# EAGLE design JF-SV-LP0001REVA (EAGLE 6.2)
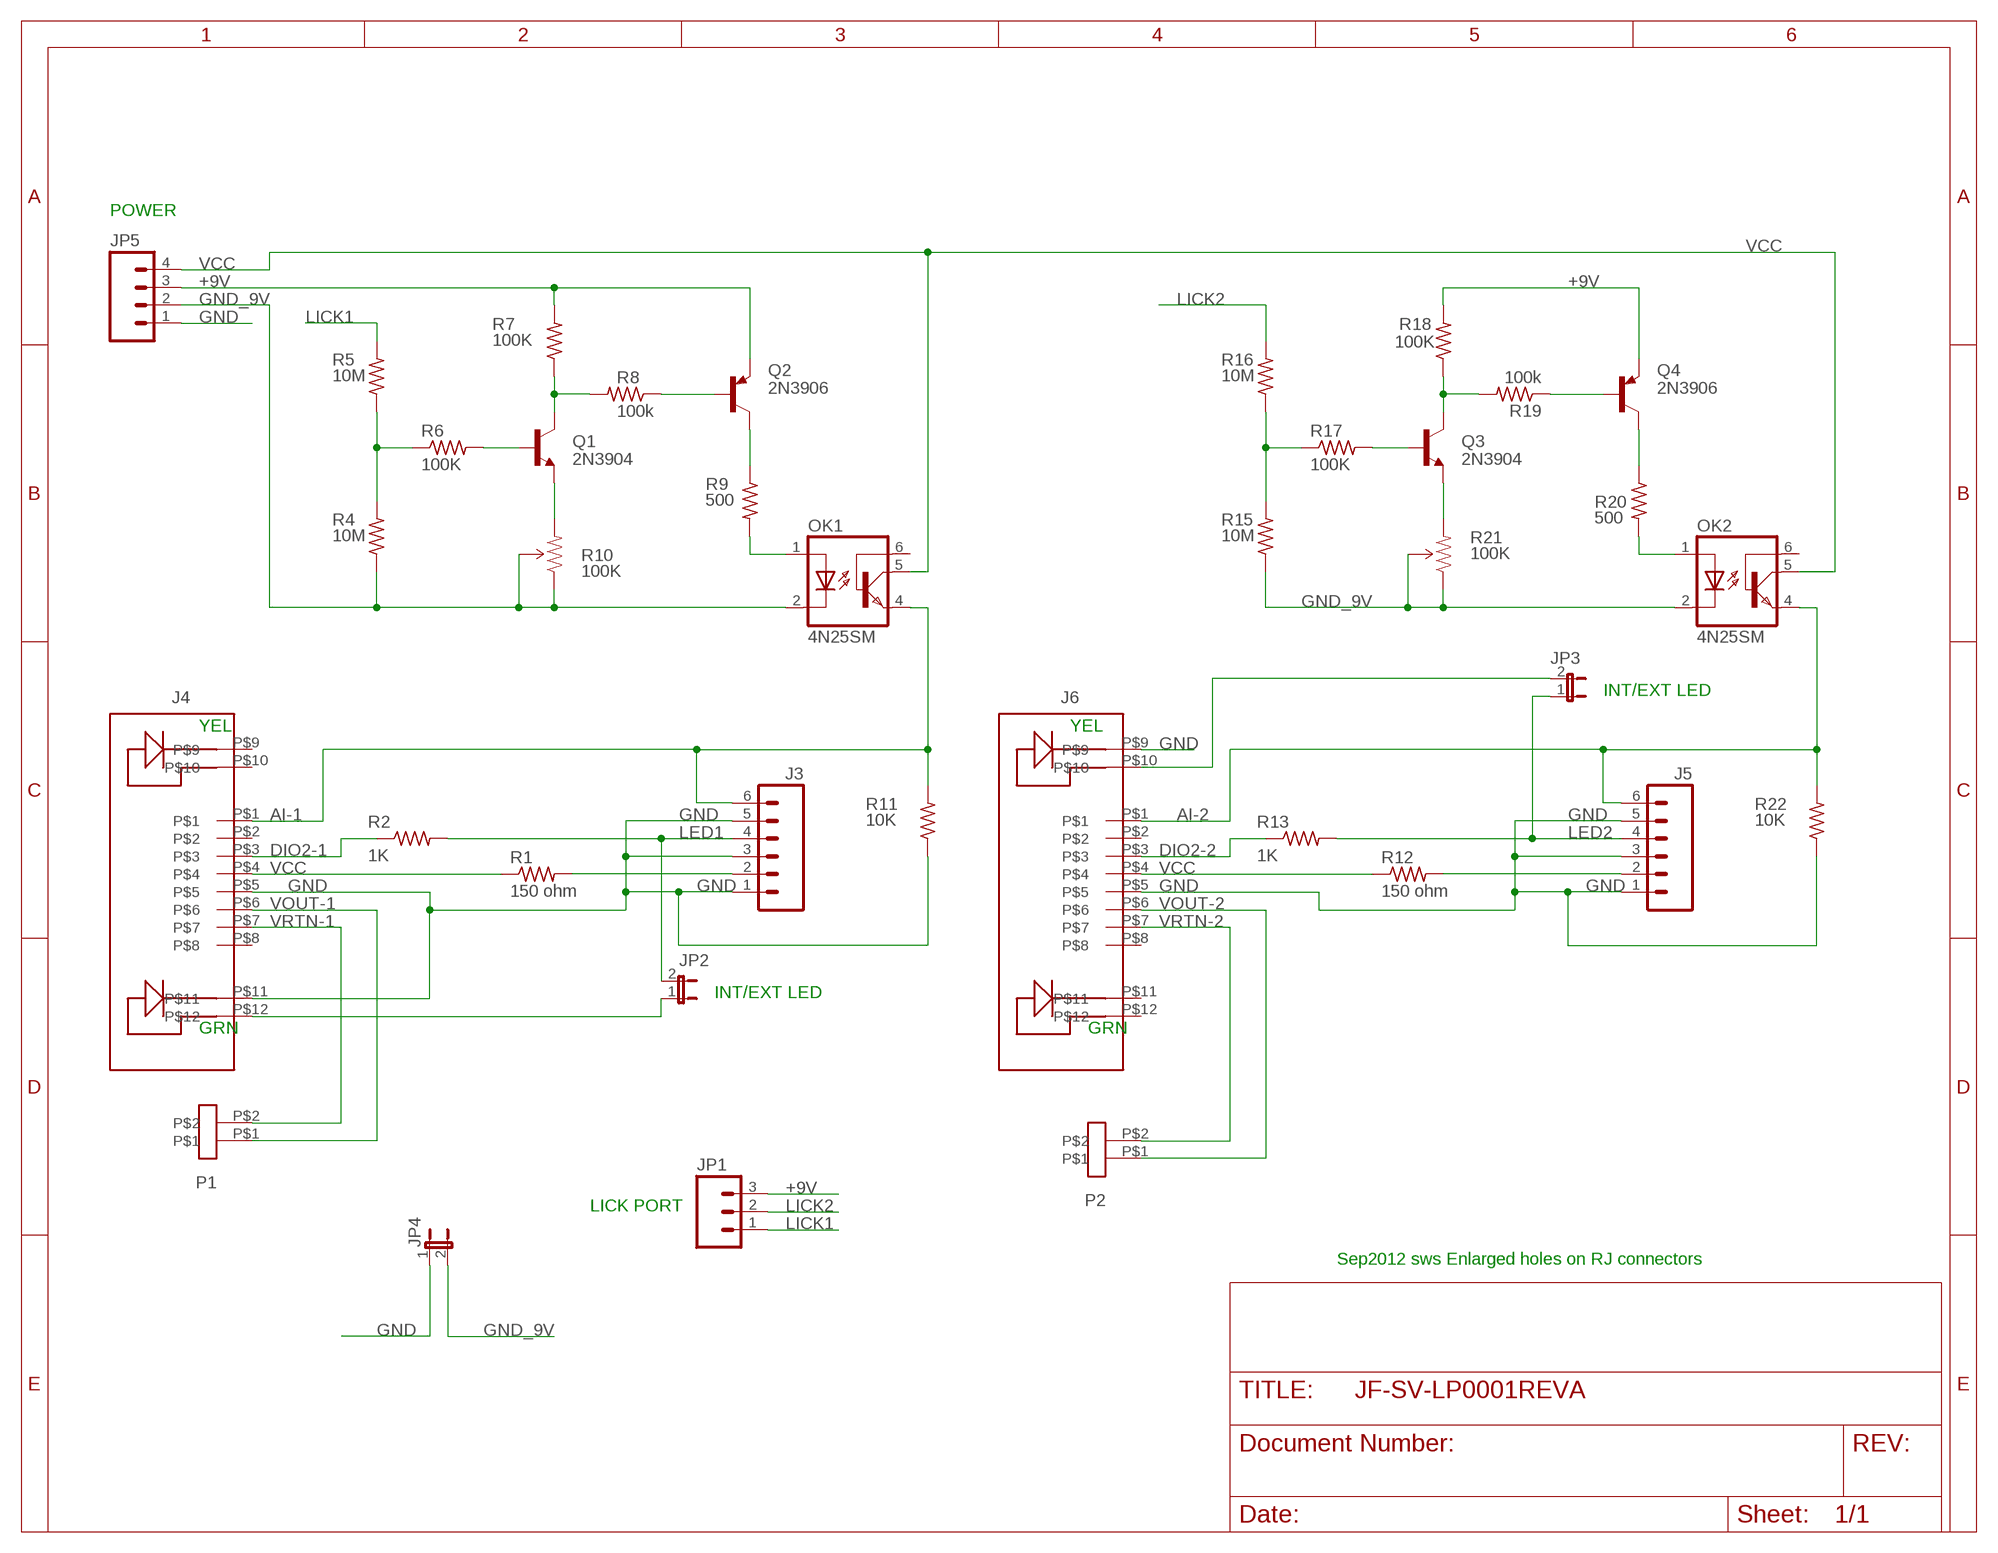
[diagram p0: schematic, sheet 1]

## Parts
J3  M063.5MM-6  [SCREWTERMINAL-3.5MM-6]
J4  RJ45_LED  [RJ45_LED]
J5  M063.5MM-6  [SCREWTERMINAL-3.5MM-6]
J6  RJ45_LED  [RJ45_LED]
JP1  M03POLAR  [MOLEX-1X3]
JP2  JP1E  [JP1]
JP3  JP1E  [JP1]
JP4  JUMPER-2PTH  [1X02]
JP5  M04POLAR  [MOLEX-1X4]
OK1  4N25SM  [DIL6-SMD]
OK2  4N25SM  [DIL6-SMD]
P1  CON2MICRO-FIT  [MICRO-FIT-2-RA]
P2  CON2MICRO-FIT  [MICRO-FIT-2-RA]
Q1  2N3904  MMBT3904LT1-NPN-SOT23-BEC  [SOT23-BEC]
Q2  2N3906  MMBT3906LT1-PNP-SOT23-BEC  [SOT23-BEC]
Q3  2N3904  MMBT3904LT1-NPN-SOT23-BEC  [SOT23-BEC]
Q4  2N3906  MMBT3906LT1-PNP-SOT23-BEC  [SOT23-BEC]
R1  150 ohm  RESISTOR_SM0805S  [0805S]
R2  1K  RESISTOR_SM0805S  [0805S]
R4  10M  RESISTOR_SM0805S  [0805S]
R5  10M  RESISTOR_SM0805S  [0805S]
R6  100K  RESISTOR_SM0805S  [0805S]
R7  100K  RESISTOR_SM0805S  [0805S]
R8  100k  RESISTOR_SM0805S  [0805S]
R9  500  RESISTOR_SM0805S  [0805S]
R10  100K  TRIMPOTPTH  [TRIM_POT_PTH]
R11  10K  RESISTOR_SM0805S  [0805S]
R12  150 ohm  RESISTOR_SM0805S  [0805S]
R13  1K  RESISTOR_SM0805S  [0805S]
R15  10M  RESISTOR_SM0805S  [0805S]
R16  10M  RESISTOR_SM0805S  [0805S]
R17  100K  RESISTOR_SM0805S  [0805S]
R18  100K  RESISTOR_SM0805S  [0805S]
R19  100k  RESISTOR_SM0805S  [0805S]
R20  500  RESISTOR_SM0805S  [0805S]
R21  100K  TRIMPOTPTH  [TRIM_POT_PTH]
R22  10K  RESISTOR_SM0805S  [0805S]

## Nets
+9V: JP1.3 JP5.3 Q2.E Q4.E R7.2 R18.2
AI-1: J3.6 J4.P$1 OK1.4(EMI) R11.2
AI-2: J5.6 J6.P$1 OK2.4(EMI) R22.2
DIO2-1: J4.P$3 R2.1
DIO2-2: J6.P$3 R13.1
GND: J3.1 J3.3 J3.5 J4.P$5 J4.P$11 J5.1 J5.3 J5.5 J6.P$5 J6.P$9 JP4.1 JP5.1 R11.1 R22.1
GND_9V: JP4.2 JP5.2 OK1.2(C) OK2.2(C) R4.1 R10.1(CCW) R10.2(WIPER) R15.1 R21.1(CCW) R21.2(WIPER)
LED1: J3.4 JP2.2 R2.2
LED2: J5.4 JP3.1 R13.2
LICK1: JP1.1 R5.2
LICK2: JP1.2 R16.2
N$1: J3.2 R1.2
N$3: OK1.1(A) R9.2
N$8: J4.P$12 JP2.1
N$12: R4.2 R5.1 R6.1
N$13: Q1.B R6.2
N$14: Q1.E R10.3(CW)
N$15: Q1.C R7.1 R8.2
N$16: Q2.B R8.1
N$18: Q2.C R9.1
N$19: J6.P$10 JP3.2
N$21: J5.2 R12.2
N$23: R15.2 R16.1 R17.1
N$24: Q3.B R17.2
N$25: Q3.E R21.3(CW)
N$26: Q3.C R18.1 R19.2
N$27: Q4.B R19.1
N$32: OK2.1(A) R20.2
N$33: Q4.C R20.1
VCC: J4.P$4 J6.P$4 JP5.4 OK1.5(COL) OK2.5(COL) R1.1 R12.1
VOUT-1: J4.P$6 P1.P$1
VOUT-2: J6.P$6 P2.P$1
VRTN-1: J4.P$7 P1.P$2
VRTN-2: J6.P$7 P2.P$2
Unconnected: J4.P$2 J4.P$8 J4.P$9 J4.P$10 J6.P$2 J6.P$8 J6.P$11 J6.P$12 OK1.6(BAS) OK2.6(BAS)

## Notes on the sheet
- POWER
- INT/EXT LED
- YEL | YEL
- INT/EXT LED
- GRN | GRN
- LICK PORT
- Sep2012 sws Enlarged holes on RJ connectors

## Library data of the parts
J3 J5 = SparkFun:M06: Header 6 Standard 6-pin 0.1" header. Use with straight break away headers (SKU : PRT-00116), right angle break away headers (PRT-00553), swiss pins (PRT-00743), machine pins (PRT-00117), and female headers (PRT-00115). Molex polarized connector foot print use with SKU : PRT-08094 with associated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
J4 J6 = SteveS:RJ45_LED
JP1 = SparkFun:M03: Header 3 Standard 3-pin 0.1" header. Use with straight break away headers (SKU : PRT-00116), right angle break away headers (PRT-00553), swiss pins (PRT-00743), machine pins (PRT-00117), and female headers (PRT-00115). Molex polarized connector foot print use with SKU : PRT-08232 with associated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
JP2 JP3 = jumper:JP1E: JUMPER
JP4 = SparkFun:JUMPER-2: Jumper
JP5 = SparkFun:M04: Header 4 Standard 4-pin 0.1" header. Use with straight break away headers (SKU : PRT-00116), right angle break away headers (PRT-00553), swiss pins (PRT-00743), machine pins (PRT-00117), and female headers (PRT-00115). Molex polarized connector foot print use with SKU : PRT-08231 with associated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
OK1 OK2 = optocoupler:4N*?M: General Purpose 6-Pin Phototransistor Optocouplers Source: http://www.fairchildsemi.com/ds/4N/4N35-M.pdf; MF: FAIRCHILD SEMICONDUCTOR; MPN: 4N25SM; OC_FARNELL: 1021152; OC_NEWARK: 34C2020
P1 P2 = SteveS:CON2
Q1 Q3 = transistor-neu-to92:*-NPN-: NPN Transistror
Q2 Q4 = transistor:*-PNP-: PNP Transistror
R1 R2 R4-R9 R11-R13 R15-R20 R22 = SteveS:RESISTOR_SM
R10 R21 = SparkFun:TRIMPOT

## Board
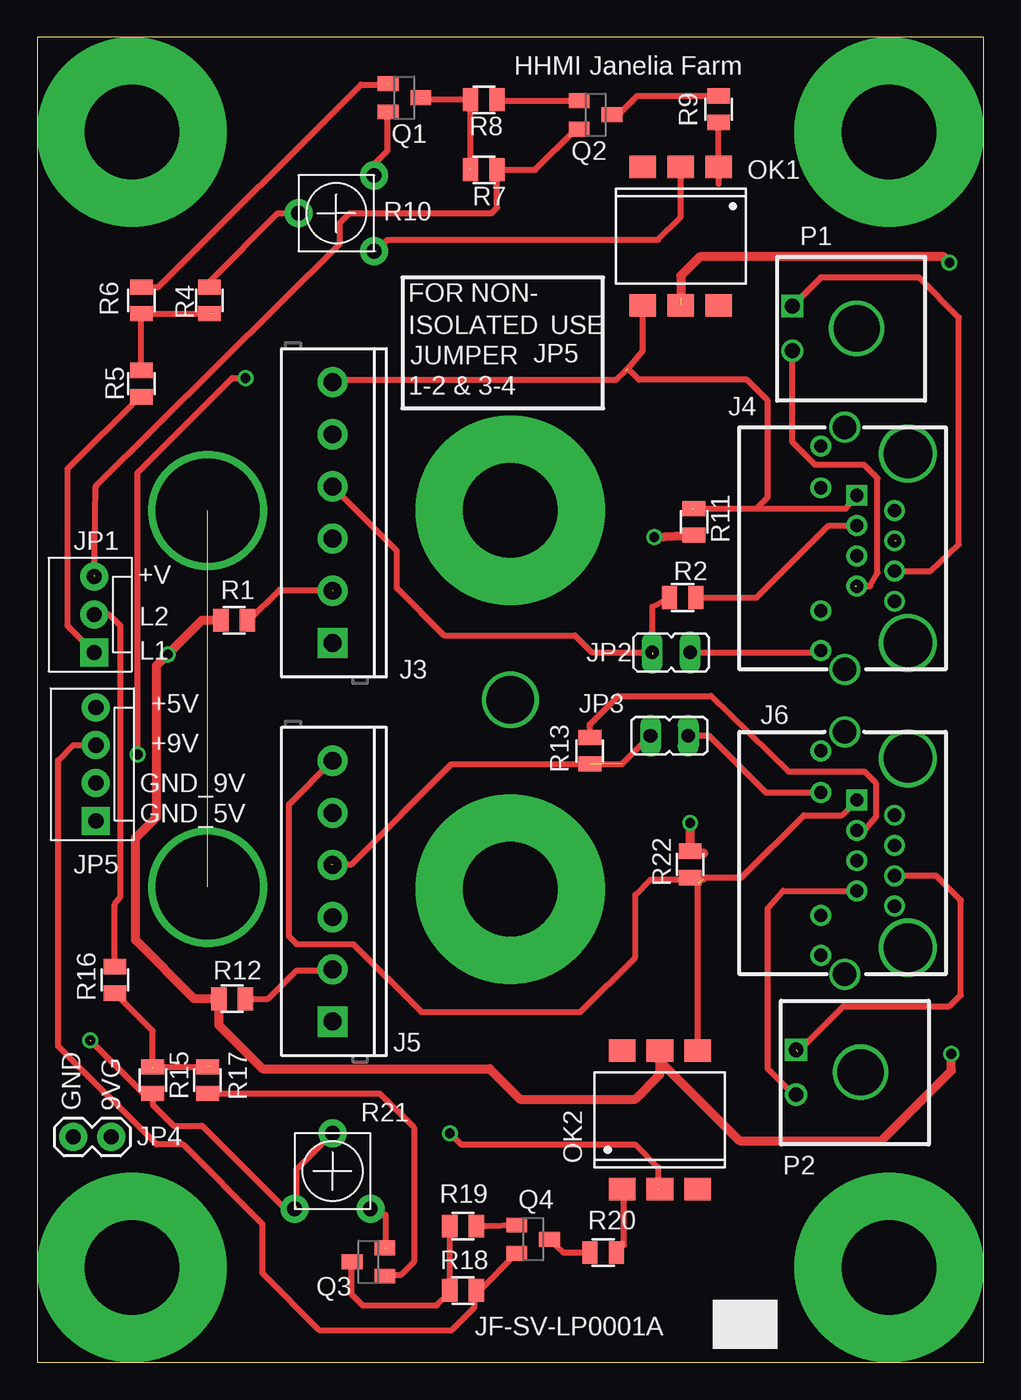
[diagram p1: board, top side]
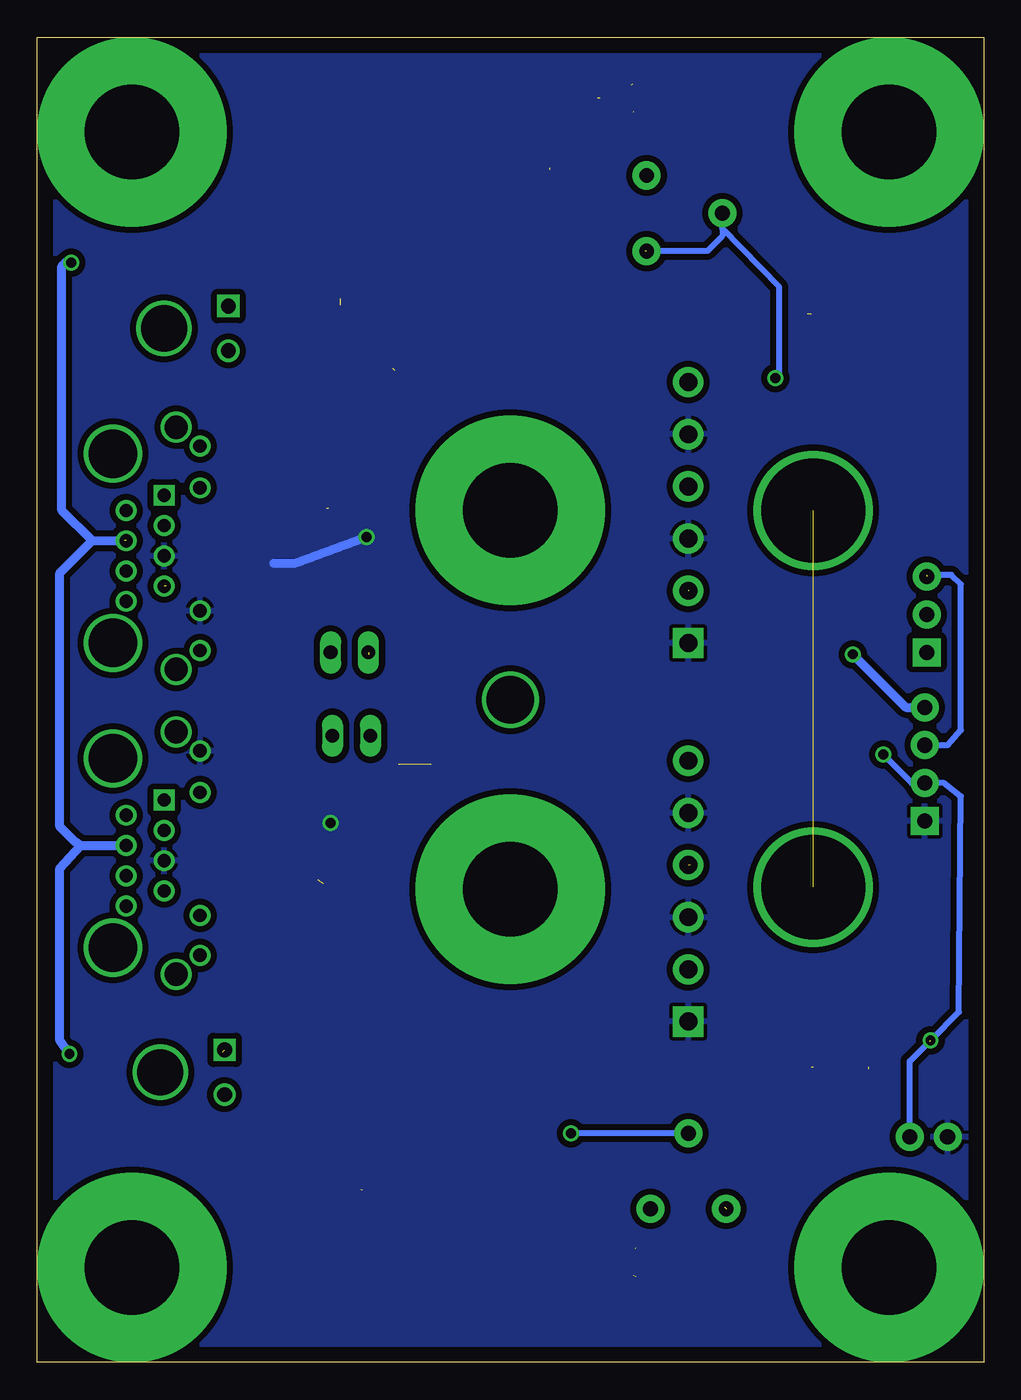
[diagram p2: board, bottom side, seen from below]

Size 63.5 x 88.9 mm. Coordinates in mm from the lower left corner, seen from the top.
Outline: 63.5,0 63.5,88.9 0,88.9 0,0 63.5,0
Copper layers (1*16): Top 0.035mm / dielectric 1.5mm / Bottom 0.035mm
Design rules: minimum track width 10mil, minimum drill 24mil, track to track 8mil, track to pad 8mil, pad to pad 8mil, via to via 8mil, smd to smd 8mil, copper to edge 40mil, drill to drill 8mil, minimum pad ring 10mil, minimum via ring 8mil, stop-mask expansion 4mil, vias tented up to drill 0mil, thermal gap 10mil

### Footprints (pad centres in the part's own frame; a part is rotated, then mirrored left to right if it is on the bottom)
SCREWTERMINAL-3.5MM-6 = drill 1.2 pad 2.032 square: 1 0,0 | drill 1.2 pad 2.032: 2 3.5,0; 3 7,0; 4 10.5,0; 5 14,0; 6 17.5,0
RJ45_LED = drill 3.251 pad 3.251: A -6.35,0; B 6.35,0 | drill 0.889 square: P$1 3.556,3.429 | drill 0.889: P$2 2.54,0.889; P$3 1.524,3.429; P$4 0.508,0.889; P$5 -0.508,3.429; P$6 -1.524,0.889; P$7 -2.54,3.429; P$8 -3.556,0.889; P$9 6.858,5.842; P$10 4.064,5.842; P$11 -4.191,5.842; P$12 -6.858,5.842 | drill 1.575 pad 2.083: P$13 8.128,4.242; P$14 -8.128,4.242
MOLEX-1X3 = drill 1.016 pad 1.88 square: 1 0,0 | drill 1.016 pad 1.88: 2 2.54,0; 3 5.08,0
JP1 = drill 0.914 long: 1 0,-1.27; 2 0,1.27
1X02 = drill 1.016 pad 1.88: 1 0,0; 2 2.54,0
MOLEX-1X4 = drill 1.016 pad 1.88 square: 1 0,0 | drill 1.016 pad 1.88: 2 2.54,0; 3 5.08,0; 4 7.62,0
DIL6-SMD = smd 1.78 x 1.52: 1 -2.54,-4.645; 2 0,-4.645; 3 2.54,-4.645; 4 2.54,4.645; 5 0,4.645; 6 -2.54,4.645
MICRO-FIT-2-RA = drill 3.099: A 1.499,4.318 | drill 0.991 square: P$1 0,0 | drill 0.991: P$2 2.997,0
SOT23-BEC = smd 1 x 1.4: B -0.95,-1.1; C 0,1.1; E 0.95,-1.1
0805S = smd 1.016 x 1.524: 1 -0.889,0; 2 0.889,0
TRIM_POT_PTH = drill 1 pad 1.88: 1 -2.54,-2.54; 2 0,2.54; 3 2.54,-2.54

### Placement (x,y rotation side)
J3  19.81,48.26 90 top
J4  58.42,54.61 90 top
J5  19.81,22.86 90 top
J6  58.42,34.16 90 top
JP1  3.81,47.62 90 top
JP2  42.55,47.62 90 top
JP3  42.42,42.04 270 top
JP4  2.41,15.11 0 top
JP5  3.94,36.32 90 top
OK1  43.18,75.56 180 top
OK2  41.78,16.26 0 top
P1  50.67,70.87 270 top
P2  50.93,20.95 270 top
Q1  24.64,84.84 270 top
Q2  37.47,83.69 270 top
Q3  22.23,6.73 90 top
Q4  33.27,8.26 270 top
R1  13.21,49.78 0 top
R2  43.31,51.31 180 top
R4  11.56,71.25 270 top
R5  6.99,65.66 270 top
R6  6.99,71.25 90 top
R7  29.97,80.01 0 top
R8  29.97,84.71 180 top
R9  45.72,84.07 270 top
R10  20.07,77.09 90 top
R11  44.07,56.39 90 top
R12  13.08,24.38 0 top
R13  37.08,41.02 270 top
R15  7.75,18.92 90 top
R16  5.21,25.65 90 top
R17  11.43,18.92 270 top
R18  28.57,4.83 0 top
R19  28.57,9.14 180 top
R20  37.97,7.37 0 top
R21  19.81,12.83 0 top
R22  43.81,33.4 270 top

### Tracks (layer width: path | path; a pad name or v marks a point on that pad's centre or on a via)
+9V  (1 unrouted)
  Top 0.406: Q2.E 36.13,82.74 33.4,80.01 R7.2 30.86,77.47 30.48,77.09 20.95,77.09 20.32,76.45 20.32,75.06 3.94,58.8 JP1.3 | Q4.E 29.65,4.76 R18.2 29.34,3.81 29.34,3.68 27.81,2.16 18.92,2.16 15.11,5.97 15.11,9.27 9.78,14.61 8,14.61 1.4,21.21 1.4,40.39 2.41,41.4 JP5.3
  Bottom 0.406: JP5.3 2.41,41.4 1.52,42.42 1.52,52.2 2.16,52.83 3.81,52.83
AI-1  (2 unrouted)
  Top 0.406: J4.P$1 54.23,57.28 48.26,57.28 | J3.6 19.96,65.91 38.86,65.91 39.5,66.55 | OK1.4 40.64,67.87 39.62,66.67 40.39,65.91 47.62,65.91 49.02,64.52 49.02,58.04 48.26,57.28 | 43.94,57.28 48.26,57.28
AI-2  (1 unrouted)
  Top 0.406: J5.6 16.89,37.44 16.89,28.57 17.4,28.07 21.21,28.07 25.78,23.5 36.45,23.5 40.13,27.18 40.13,31.37 41.15,32.38 44.7,32.38 44.83,32.51 47.24,32.51 51.44,36.7 53.98,36.7 J6.P$1 | OK2.4 44.32,32.13 R22.2
DIO2-1
  Top 0.406: J4.P$3 53.09,56.13 48.26,51.31 R2.1
DIO2-2
  Top 0.406: R13.1 37.08,42.8 38.99,44.7 45.21,44.7 50.42,39.62 55.5,39.62 56.26,38.86 56.26,36.58 55.5,35.69 J6.P$3
GND  (via drill 0.66)
  Top 0.61: 44.2,55.37 R11.1 v41.4,55.37 | 44.7,34.16 R22.1 v43.81,36.2
  Bottom 0.61: v41.4,55.37 46.23,53.59 47.62,53.59
  pour Bottom (isolate 0.406): 0.89,88.01 0.89,0.64 62.61,0.64 62.61,88.01
GND_9V  (via drill 0.66)  (4 unrouted)
  Top 0.406: R21.1 16.64,10.29 11.05,15.88 9.14,15.88 7.75,17.27 R15.1 7.11,18.03 v3.56,21.59 | R21.2 17.4,12.95 17.4,10.41 | v27.69,15.37 28.45,14.61 40.13,14.61 41.66,13.08 41.66,11.56 | OK1.2 43.18,76.83 41.66,75.31 23.5,75.31 22.73,74.55 | R4.1 11.56,72.52 16.13,77.09 R10.2 | v6.73,40.77 6.73,59.69 13.08,66.04 v13.97,66.04
  Bottom 0.406: v3.56,21.59 1.65,23.5 1.52,37.97 2.67,38.86 JP5.2 4.83,38.86 v6.73,40.77 | R21.2 v27.69,15.37 | R10.1 18.54,74.55 17.53,75.56 17.53,76.07 | v13.97,66.04 13.72,66.29 13.72,72.14 17.53,76.07 | 17.53,76.07 R10.2 | JP4.2 4.95,20.19 3.62,21.53
LED1  (1 unrouted)
  Top 0.406: J3.4 24.13,54.44 24.13,51.94 27.3,48.77 36.07,48.77 37.21,47.62 JP2.2 | R2.2 41.27,50.67 41.27,47.5
LED2  (2 unrouted)
  Top 0.406: JP3.1 39.24,40.13 27.81,40.13 21.08,33.4 19.68,33.4
LICK1
  Top 0.406: JP1.1 2.03,49.4 2.03,59.94 6.86,64.77 R5.2
LICK2
  Top 0.406: R16.2 5.21,30.73 5.59,31.24 5.59,49.4 4.83,50.16 JP1.2
N$1  (1 unrouted)
  Top 0.406: R1.2 14.22,49.78 16.26,51.82 19.81,51.82 19.94,51.69
N$3
  Top 0.406: R9.2 OK1.1 45.72,79.07
N$4  (via drill 3.17)
  other vias: 31.75,44.45
N$5  (via drill 6.35 pad 12.7)
  other vias: 6.35,6.35
N$6  (via drill 6.35 pad 12.7)
  other vias: 57.15,6.35
N$7  (via drill 6.35 pad 12.7)
  other vias: 57.15,82.55
N$8
  Top 0.406: J4.P$12 51.94,47.62 JP2.1
N$9  (via drill 6.35 pad 12.7)
  other vias: 31.75,57.15
N$10  (via drill 6.35 pad 12.7)
  other vias: 31.75,31.75
N$12  (1 unrouted)
  Top 0.406: R5.1 R6.1 11.81,70.36
N$13  (1 unrouted)
  Top 0.406: R6.2 8.13,72.14 21.72,85.72 23.62,85.72
N$14  (1 unrouted)
  Top 0.406: R10.3 22.61,80.39 23.5,81.28 23.5,83.95
N$15  (2 unrouted)
  Top 0.406: 29.08,80.14 R8.2 26.04,84.71 25.91,84.84
N$16
  Top 0.406: Q2.B 30.93,84.64 R8.1
N$17  (via drill 6.35 pad 12.7)
  other vias: 6.35,82.55
N$18
  Top 0.406: Q2.C 38.99,83.69 40.26,84.96 R9.1 45.85,84.84
N$19
  Top 0.406: JP3.2 45.09,42.04 48.9,38.23 J6.P$10 52.58,38.1
N$21
  Top 0.406: R12.2 15.49,24.38 17.4,26.29 19.74,26.29 J5.2
N$23  (2 unrouted)
  Top 0.406: R16.1 7.75,22.23 7.75,19.68 7.87,19.81 11.56,19.81
N$24  (1 unrouted)
  Top 0.406: R17.2 22.99,18.03 25.27,15.75 25.27,6.73 24.38,5.84 23.5,5.84
N$25  (1 unrouted)
  Top 0.406: R21.3 22.73,9.91 23.37,9.91 23.37,7.62
N$26
  Top 0.406: R19.2 R18.1 27.69,4.7 26.8,3.81 21.84,3.81 21.08,4.57 21.08,6.18 Q3.C
N$27
  Top 0.406: Q4.B 30.2,9.14 R19.1
N$32
  Top 0.406: OK2.1 39.37,11.48 39.37,7.87 R20.2
N$33
  Top 0.406: R20.1 35.31,7.37 Q4.C
NC2  (via drill 6.99)  (1 unrouted)
  other vias: 11.43,57.15 11.43,31.88
VCC  (via drill 0.66)  (2 unrouted)
  Top 0.61: R1.1 11.05,49.78 v8.76,47.5 8,46.74 8,36.58 6.6,35.18 6.6,28.32 10.54,24.38 R12.1 12.19,22.61 15.11,19.68 30.35,19.68 32.38,17.65 40.13,17.65 41.78,19.3 OK2.5 41.66,20.77 41.66,20.32 47.12,14.86 56.64,14.86 61.34,19.56 v61.34,20.7 | v61.21,73.79 60.83,74.17 44.45,74.17 43.18,72.9 43.18,71.37
  Bottom 0.61: v8.76,47.5 5.21,43.94 JP5.4 | v61.34,20.7 61.98,21.59 61.98,33.15 60.58,34.67 | 60.58,34.67 J6.P$4 | 60.58,34.67 60.96,34.92 61.98,35.94 61.98,52.96 59.82,55.12 | 59.82,55.12 57.66,55.12 | 59.82,55.12 61.85,57.15 61.85,73.53 61.59,73.79 v61.21,73.79
VOUT-1
  Top 0.406: P1.P$1 52.58,72.77 59.18,72.77 61.85,70.1 61.85,54.86 59.94,53.09 J4.P$6
VOUT-2  (1 unrouted)
  Top 0.406: J6.P$6 60.33,32.64 61.98,30.99 61.98,24.64 61.21,23.88 54.1,23.88 51.05,20.83
VRTN-1  (1 unrouted)
  Top 0.406: P1.P$2 50.67,61.72 52.2,60.2 55.5,60.2 56.39,59.31 56.39,52.96 55.88,52.07 54.86,52.07
VRTN-2
  Top 0.406: P2.P$2 50.75,17.96 49.02,19.68 49.02,30.48 50.04,31.62 J6.P$7

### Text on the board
tPlace: HHMI Janelia Farm | P1 | FOR | NON- | ISOLATED | USE | JUMPER | JP5 | 1-2 & 3-4 | J4 | JP1 | +V | L2 | L1 | +5V | J6 | +9V | GND_9V | GND_5V | JP5 | GND | 9VG | P2 | JF-SV-LP0001A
